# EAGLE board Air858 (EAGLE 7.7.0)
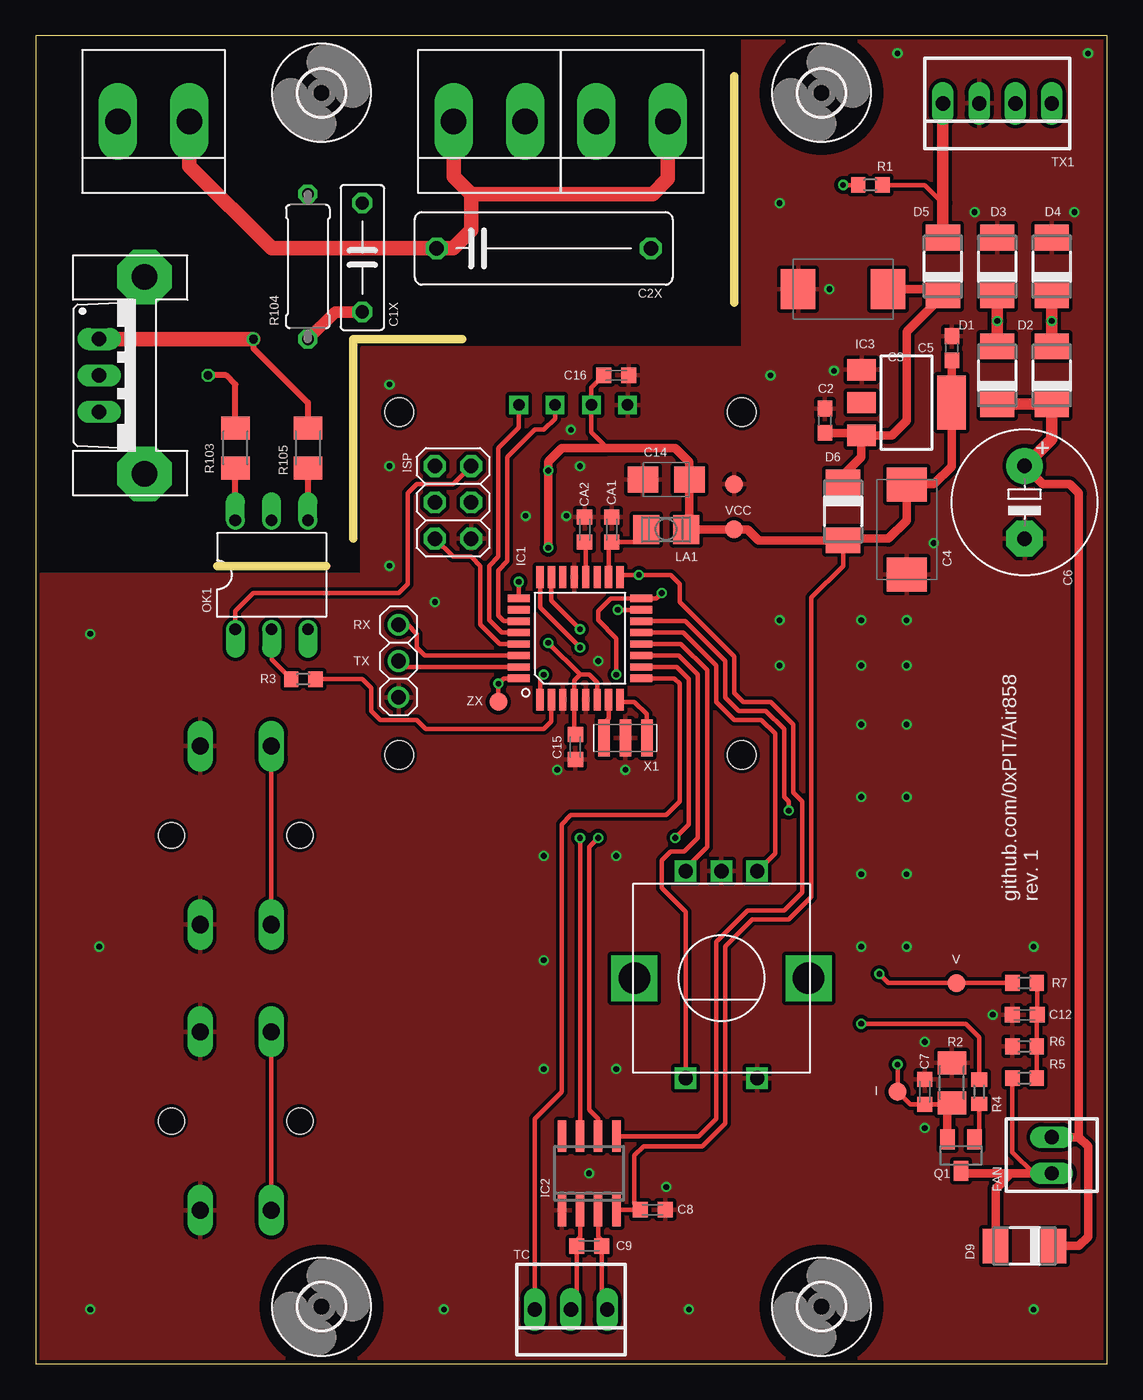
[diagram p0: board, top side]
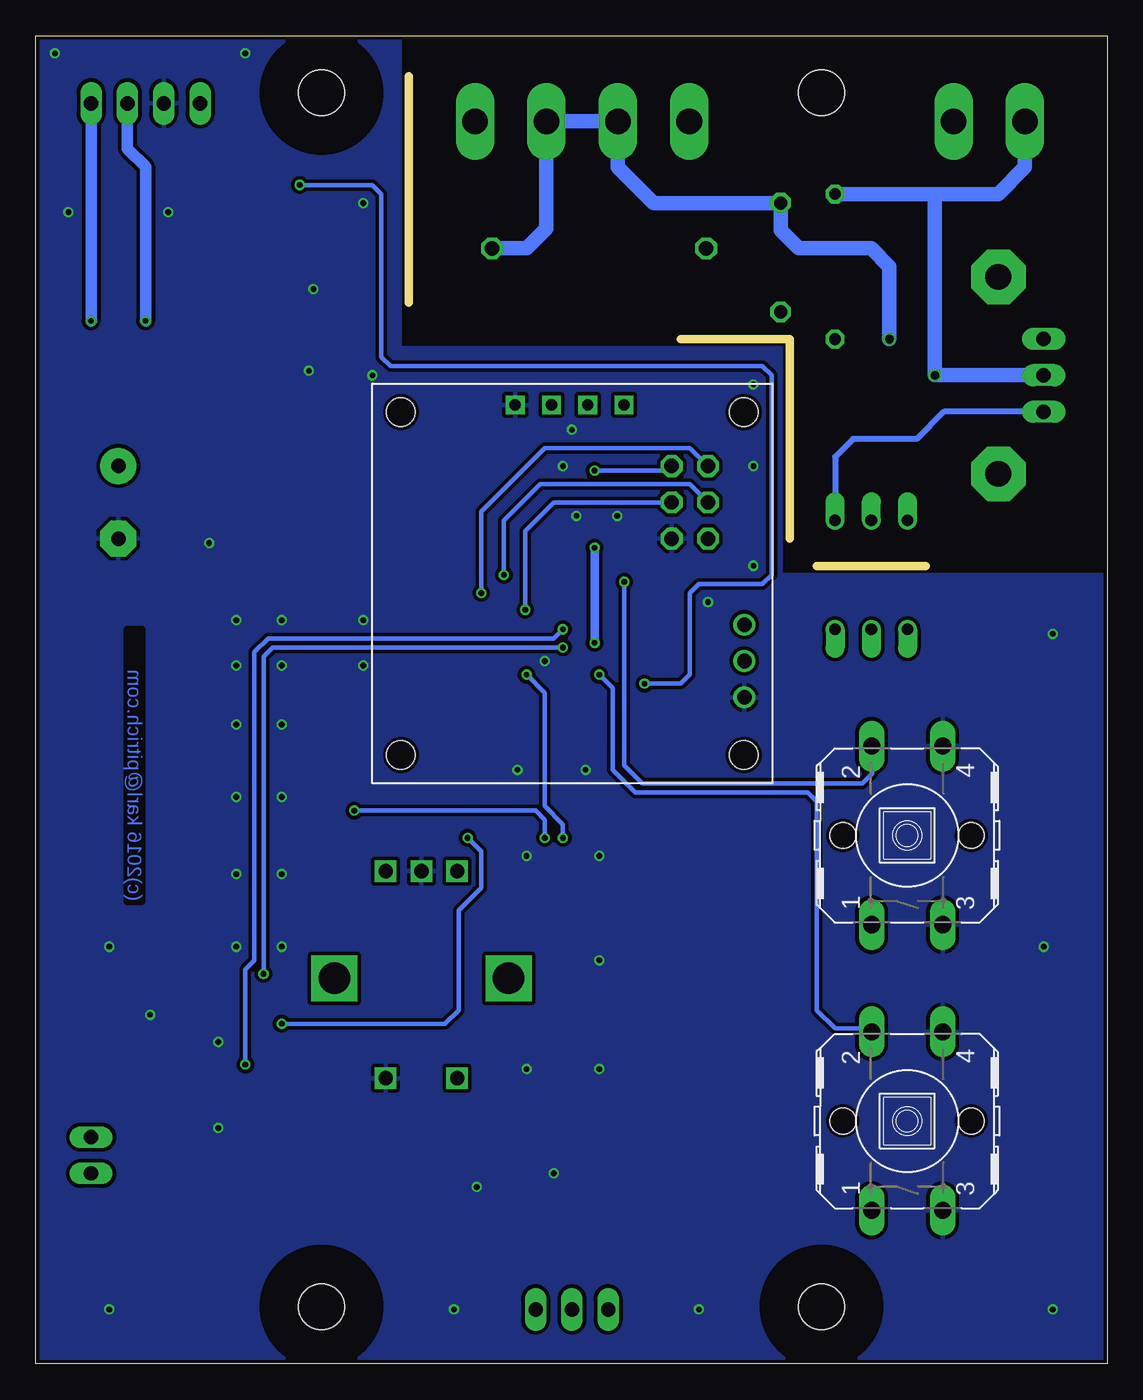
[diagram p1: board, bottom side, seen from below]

Size 75 x 93 mm. Coordinates in mm from the lower left corner, seen from the top.
Outline: 0,0 75,0 75,93 0,93 0,0
Copper layers (1*16): Top 0.035mm / dielectric 1.5mm / Bottom 0.035mm
Design rules "dirt_cheap_dirty_boards.v1": minimum track width 5mil, minimum drill 12mil, track to track 5mil, track to pad 5mil, pad to pad 5mil, via to via 5mil, smd to smd 0mil, copper to edge 10mil, drill to drill 10mil, minimum pad ring 10mil, minimum via ring 6mil, stop-mask expansion 2mil, vias tented up to drill 25mil, thermal gap 10mil
Milling: 4 lines

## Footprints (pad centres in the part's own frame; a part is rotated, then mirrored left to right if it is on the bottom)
B1,27 = smd 1.27 x 1.27: TP 0,0
C075-032X103 = drill 0.914 octagon: 1 -3.81,0; 2 3.81,0
C0603 = smd 1.1 x 1: 1 -0.85,0; 2 0.85,0
C150-054X183 = drill 1.016 octagon: 1 -7.493,0; 2 7.493,0
SMC_E = smd 2.4 x 2.8: + -3.15,0; - 3.15,0
E5-10,5 = drill 1.016 pad 2.54: + -2.54,0 | drill 1.016 pad 2.54 octagon: - 2.54,0
C0603K = smd 1.05 x 1.08: 1 -0.875,0; 2 0.875,0
B/3528-21W = smd 2.15 x 1.8: + 1.625,0; - -1.625,0
DO-214AC = smd 1.8 x 2.4: A 2.025,0; C -2.025,0
22-23-2021 = drill 1 long: 1 -1.27,0; 2 1.27,0
2POL5MM = drill 1.8 long: 1 -2.5,0; 2 2.5,0
QFP32 = smd 0.508 x 1.524: 1 -2.8,-4.293; 2 -2,-4.293; 3 -1.2,-4.293; 4 -0.4,-4.293; 5 0.4,-4.293; 6 1.2,-4.293; 7 2,-4.293; 8 2.8,-4.293; 17 2.8,4.293; 18 2,4.293; 19 1.2,4.293; 20 0.4,4.293; 21 -0.4,4.293; 22 -1.2,4.293; 23 -2,4.293; 24 -2.8,4.293 | smd 1.524 x 0.508: 9 4.293,-2.8; 10 4.293,-2; 11 4.293,-1.2; 12 4.293,-0.4; 13 4.293,0.4; 14 4.293,1.2; 15 4.293,2; 16 4.293,2.8; 25 -4.293,2.8; 26 -4.293,2; 27 -4.293,1.2; 28 -4.293,0.4; 29 -4.293,-0.4; 30 -4.293,-1.2; 31 -4.293,-2; 32 -4.293,-2.8
SOIC8 = smd 0.6 x 2.2: 1 -1.905,-2.6; 2 -0.635,-2.6; 3 0.635,-2.6; 4 1.905,-2.6; 5 1.905,2.6; 6 0.635,2.6; 7 -0.635,2.6; 8 -1.905,2.6
SOT223 = smd 1.5 x 2: 1 -2.3,-3.15; 2 0,-3.15; 3 2.3,-3.15 | smd 3.8 x 2: 4 0,3.15
2X03 = drill 1.016 octagon: 1 -2.54,-1.27; 2 -2.54,1.27; 3 0,-1.27; 4 0,1.27; 5 2.54,-1.27; 6 2.54,1.27
1X03 = drill 1.016: 1 -2.54,0; 2 0,0; 3 2.54,0
L3225P = smd 1.8 x 2: 1 -1.4,0; 2 1.4,0
DIL06 = drill 0.813 offset: 1 -2.54,-3.81; 2 0,-3.81; 3 2.54,-3.81; 4 2.54,3.81; 5 0,3.81; 6 -2.54,3.81
SSD1306-IIC = drill 0.8 square: GND 10,26.5; SCL 15.08,26.5; SDA 17.62,26.5; VCC 12.54,26.5 | hole 2: 2,2; 26,26; 26,2; 2,26
SOT23 = smd 1 x 1.4: 1 -0.95,-1.1; 2 0.95,-1.1; 3 0,1.1
R0603 = smd 1 x 1.1: 1 -0.85,0; 2 0.85,0
M1206 = smd 1.6 x 2: 1 -1.4,0; 2 1.4,0
0309/10 = drill 0.813 octagon: 1 -5.08,0; 2 5.08,0
B3F-40XX = drill 1.194 long: 1 -6.248,2.489; 2 6.248,2.489; 3 -6.248,-2.489; 4 6.248,-2.489 | hole 1.803: 0,-4.496; 0,4.496
ALPS_EC12E_SW = drill 1 square: A -2.5,-7.5; B 2.5,-7.5; C 0,-7.5; D -2.5,7; E 2.5,7 | drill 2.2 square: GND1 -6.1,0; GND2 6.1,0
TO220BV = drill 1.016 long: G 2.54,-2.54; T1 -2.54,-2.54; T2 0,-2.54
22-23-2031 = drill 1 long: 1 -2.54,0; 2 0,0; 3 2.54,0
22-23-2041 = drill 1 long: 1 -3.81,0; 2 -1.27,0; 3 1.27,0; 4 3.81,0
3,2 = hole 3.2: 0,0
HEATSINK17X7.5TO220 = drill 1.8 pad 3.81 octagon: P$1 -6.9,0; P$2 6.9,0
CSTCR6M = smd 0.8 x 2.6: 1 -1.5,0; 2 0,0; 3 1.5,0

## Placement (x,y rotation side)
0V  PTR1B1,27  [B1,27]  48.9,61.59 0 top
C1X  10n  [C075-032X103]  22.86,77.47 270 top
C2  100~n  [C0603]  55.24,66.04 90 top
C2X  100n  [C150-054X183]  35.56,78.11 0 top
C3  220µ  [SMC_E]  56.52,75.25 180 top
C4  220µ  [SMC_E]  60.96,58.42 270 top
C5  100n  [C0603]  64.14,71.12 90 top
C6  470µ  [E5-10,5]  69.22,60.33 270 top
C7  100n  [C0603K]  62.23,19.05 90 top
C8  100n  [C0603K]  43.18,10.79 0 top
C9  100n  [C0603K]  38.73,8.26 180 top
C12  100n  [C0603K]  69.22,24.45 180 top
C14  10µ  [B/3528-21W]  44.13,61.91 0 top
C15  100n  [C0603K]  37.78,43.18 270 top
C16  100n  [C0603K]  40.64,69.22 180 top
CA1  100n  [C0603K]  40.32,58.42 90 top
CA2  100n  [C0603K]  38.42,58.42 270 top
D1  [DO-214AC]  67.31,69.22 90 top
D2  [DO-214AC]  71.12,69.22 90 top
D3  [DO-214AC]  67.31,76.83 90 top
D4  [DO-214AC]  71.12,76.83 90 top
D5  [DO-214AC]  63.5,76.83 90 top
D6  [DO-214AC]  56.52,59.69 270 top
D9  [DO-214AC]  69.22,8.26 180 top
FAN  J1  [22-23-2021]  71.12,14.61 270 top
HEATER  2POL5MM  [2POL5MM]  8.26,87 0 top
I  PTR1B1,27  [B1,27]  60.33,19.05 0 top
IC1  ATMEGA168  [QFP32]  38.1,50.8 0 top
IC2  MAX31855  [SOIC8]  38.73,13.34 0 top
IC3  LD117  [SOT223]  60.96,67.31 270 top
ISP  [2X03]  29.21,60.33 270 top
JP1  [1X03]  25.4,49.21 270 top
LA1  10µ  [L3225P]  44.13,58.42 180 top
MAINS1  2POL5MM  [2POL5MM]  31.75,87 0 top
MAINS2  2POL5MM  [2POL5MM]  41.75,87 0 top
OK1  MOC3041M  [DIL06]  16.51,55.24 0 top
OLED1  [SSD1306-IIC]  51.44,40.64 0 bottom
Q1  TSM3404  [SOT23]  64.77,14.61 180 top
R1  47k  [R0603]  58.42,82.55 180 top
R2  10R  [M1206]  64.14,19.68 270 top
R3  270R  [R0603]  18.73,47.94 180 top
R4  100R  [R0603]  66.04,19.05 270 top
R5  10k  [R0603]  69.22,20 180 top
R6  1k  [R0603]  69.22,22.23 0 top
R7  10k  [R0603]  69.22,26.67 0 top
R103  360R  [M1206]  13.97,64.14 270 top
R104  51R  [0309/10]  19.05,76.83 90 top
R105  330R  [M1206]  19.05,64.14 90 top
S3  [B3F-40XX]  14,37 90 bottom
S4  [B3F-40XX]  14,17 90 bottom
SW1  EC12E_SW  [ALPS_EC12E_SW]  48,27 180 top
T1  BTA16  [TO220BV]  6.99,69.22 270 top
TC  J2  [22-23-2031]  37.47,3.81 180 top
TX1  J4  [22-23-2041]  67.31,88.27 180 top
U$1  [3,2]  20,89 0 top
U$2  [3,2]  55,89 0 top
U$3  [3,2]  20,4 0 top
U$4  [3,2]  55,4 0 top
U$5  HEATSINK17X7.5TO220  [HEATSINK17X7.5TO220]  7.62,69.22 90 top
V  PTR1B1,27  [B1,27]  64.45,26.67 0 top
VCC  PTR1B1,27  [B1,27]  48.9,58.42 0 top
X1  CSTCR6M00G53Z  [CSTCR6M]  41.27,43.81 180 top
ZX  PTR1B1,27  [B1,27]  32.38,46.35 0 top

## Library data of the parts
0V I V VCC ZX = testpad
C1X C2 C2X C3-C9 C12 C14-C16 CA1 CA2 LA1 R1-R7 R103-R105 = rcl
D1-D6 D9 = diode
FAN = con-molex; MF: MOLEX; MPN: 22-23-2021; OC_FARNELL: 1462926; OC_NEWARK: 25C3832
HEATER MAINS1 MAINS2 OLED1 U$5 = pit
IC1 = tidyeagle
IC2 = AlexW-Eagle-Libraries
IC3 = v-reg
ISP = pinhead
JP1 Q1 = adafruit
OK1 = optocoupler; MF: FAIRCHILD SEMICONDUCTOR; MPN: MOC3041M; OC_FARNELL: 1086677; OC_NEWARK: 78K6090
S3 S4 = switch-omron; MF: OMRON COMPONENTS USA; MPN: B3F-4000; OC_FARNELL: 176434; OC_NEWARK: 36K3105
SW1 = switch-alps; MPN: EC12E2424407; OC_FARNELL: 1520813; OC_NEWARK: 74M1068
T1 = triac
TC = con-molex; MF: MOLEX; MPN: 22-23-2031; OC_FARNELL: 1462950; OC_NEWARK: 30C0862
TX1 = con-molex; MF: MOLEX; MPN: 22-23-2041; OC_FARNELL: 1462920; OC_NEWARK: 38C0355
U$1-U$4 = holes
X1 = murata-filter; MPN: CSTCR6M00G53-R0; OC_FARNELL: 1170434; OC_NEWARK: 25M8759

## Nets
10V_AC1: D5.A R1.1 TX1.4
25V_AC1: D1.A D3.C TX1.2
25V_AC2: D2.A D4.C TX1.1
+3V3: C4.+ C5.1 C8.1 C14.+ C15.1 C16.2 D6.A IC1.4 IC1.6 IC2.4 IC3.4 ISP.2 LA1.1 OK1.1 OLED1.VCC VCC.TP
+24V: C6.+ D1.C D2.C D9.C FAN.1
AREF: CA2.2 IC1.20
AVCC: CA1.1 IC1.18 LA1.2
ENC_A: IC1.12 SW1.B
ENC_B: IC1.13 SW1.A
ENC_SW: IC1.11 SW1.E
FAN: IC1.10 R4.1
FAN-: D9.A FAN.2 Q1.3 R5.2
FAN_SENSE_I: C7.1 I.TP IC1.23 Q1.2 R2.2
FAN_SENSE_V: IC1.24 R7.1 V.TP
GND: 0V.TP C2.2 C3.- C4.- C5.2 C6.- C7.2 C8.2 C12.2 C14.- C15.2 C16.1 CA1.2 CA2.1 D3.A D4.A IC1.3 IC1.5 IC1.21 IC2.1 IC3.1 ISP.6 JP1.3 OLED1.GND R2.1 R6.1 S3.3 S3.4 S4.3 S4.4 SW1.C SW1.D TX1.3 X1.2
HEATER: IC1.2 R3.1
HEATER_DRIVE: HEATER.1 R103.1 R104.2 T1.T2
MAINS_L: C2X.1 HEATER.2 MAINS1.1 MAINS2.2
MAINS_N: C1X.1 C2X.2 MAINS1.2 MAINS2.1 R105.2 T1.T1
MISO: IC1.16 IC2.7 ISP.1
MOSI: IC1.15 ISP.4
N$1: C12.1 R5.1 R6.2 R7.2
N$3: OK1.6 R103.2
N$4: C2.1 C3.+ D5.C D6.C IC3.3
N$5: OK1.2 R3.2
N$8: OK1.4 R105.1 T1.G
N$9: C1X.2 R104.1
N$10: IC1.7 X1.3
N$11: Q1.1 R4.2
N$12: IC1.8 X1.1
REED: IC1.9 TC.3
RESET: IC1.29 ISP.5
RXD: IC1.30 JP1.1
SCK: IC1.17 IC2.5 ISP.3
SCL: IC1.27 OLED1.SCL
SDA: IC1.28 OLED1.SDA
SS: IC1.14 IC2.6
SW1: IC1.1 S4.1 S4.2
SW2: IC1.25 S3.1 S3.2
T+: C9.1 IC2.3 TC.1
T-: C9.2 IC2.2 TC.2
TXD: IC1.31 JP1.2
ZEROX: IC1.32 R1.2 ZX.TP

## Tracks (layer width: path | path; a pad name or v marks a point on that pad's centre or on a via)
10V_AC1
  Top 0.305: R1.1 62.23,82.55 63.5,81.28
  Top 0.813: D5.A 63.5,81.28 TX1.4
25V_AC1  (via drill 0.4)
  Top 0.813: D1.A v67.31,73.03 D3.C
  Bottom 0.813: TX1.2 68.58,85.09 67.31,83.82 v67.31,73.03
25V_AC2  (via drill 0.4)
  Top 0.813: D2.A v71.12,73.03 D4.C
  Bottom 0.813: TX1.1 v71.12,73.03
+3V3  (via drill 0.4)
  Top 0.305: C16.2 38.9,68.34 OLED1.VCC 38.9,65.25 40.01,64.14 | ISP.2 29.21,61.59 26.67,61.59 26.04,60.96 26.04,54.61 25.4,53.98 15.24,53.98 13.97,52.7 OK1.1 | C15.1 37.7,44.14 IC1.4 37.7,47.86 38.1,48.26 | IC1.6 39.3,47.7 38.73,48.26 38.1,48.26 | 38.1,48.26 v35.88,50.48 | IC2.4 40.7,10.79 C8.1 41.91,11.19 41.91,14.61 42.55,15.24 46.67,15.24 48.26,16.83 48.26,29.21 50.16,31.11 52.7,31.11 54.29,32.7 54.29,53.66 56.52,55.88 D6.A
  Top 0.61: v35.88,57.15 v35.88,62.55 35.88,63.18 36.83,64.14 40.01,64.14 44.77,64.14 45.76,63.15 C14.+ 45.76,58.65 LA1.1 VCC.TP 49.85,58.42 50.6,57.66 D6.A 56.63,57.78 59.69,57.78 60.96,59.05 C4.+ 60.98,61.59 62.87,61.59 64.11,62.84 IC3.4 64.11,70.25 C5.1
  Bottom 0.305: ISP.2 30.8,62.55 v35.88,62.55
  Bottom 0.61: v35.88,50.48 v35.88,57.15
+24V
  Top 0.61: 73.03,15.88 73.03,60.96 72.39,61.59 70.48,61.59 C6.+ | FAN.1 73.03,15.88 | 73.03,15.88 73.66,15.24 73.66,8.89 73.03,8.26 D9.C
  Top 0.813: D1.C D2.C 71.12,64.77 C6.+
AREF
  Top 0.305: IC1.20 38.5,57.46 CA2.2
AVCC
  Top 0.305: IC1.18 40.1,57.32 CA1.1 42.49,57.55 LA1.2
ENC_A
  Top 0.305: IC1.12 45.17,50.4 46.99,48.58 46.99,36.2 45.5,34.7 SW1.B
ENC_B
  Top 0.305: IC1.13 45.32,51.2 47.62,48.9 47.62,46.35 48.9,45.09 50.8,45.09 51.75,44.13 51.75,35.75 SW1.A
ENC_SW
  Top 0.305: IC1.11 45.02,49.6 46.35,48.26 46.35,36.83 45.4,35.88 44.45,35.88 43.81,35.24 43.81,33.34 45.5,31.65 SW1.E
FAN  (via drill 0.4)
  Top 0.305: IC1.10 44.86,48.8 45.72,47.94 45.72,37.78 v44.77,36.83 | R4.1 66.04,22.86 65.09,23.81 v57.78,23.81
  Bottom 0.305: v44.77,36.83 43.81,35.88 43.81,33.34 45.4,31.75 45.4,24.77 46.35,23.81 v57.78,23.81
FAN-
  Top 0.305: R5.2 68.36,14.82 69.85,13.34
  Top 0.61: FAN.2 69.85,13.34 68.26,13.34 | 68.26,13.34 64.94,13.34 Q1.3 | D9.A 67.19,12.26 68.26,13.34
FAN_SENSE_I  (via drill 0.4)
  Top 0.305: IC1.23 36.1,53.44 v38.1,51.44 | v60.33,20.95 I.TP 61.2,18.18 C7.1 64.05,18.18
  Top 0.61: R2.2 64.05,18.18 63.82,17.95 Q1.2
  Bottom 0.305: v38.1,51.44 38.73,50.8 58.74,50.8 59.69,49.85 59.69,28.26 60.33,27.62 v60.33,20.95
FAN_SENSE_V  (via drill 0.4)
  Top 0.305: IC1.24 35.3,52.97 v38.1,50.16 | v59.05,27.3 59.69,26.67 64.14,26.67 V.TP R7.1
  Bottom 0.305: v38.1,50.16 58.42,50.16 59.05,49.53 v59.05,27.3
GND  (via drill 0.4)
  other vias: 41.27,41.59 36.51,41.59 38.73,13.34 4.45,29.21 52.07,52.07 55.88,69.53 52.07,81.28 52.07,48.9 57.78,48.9 57.78,52.07 60.96,48.9 60.96,44.77 57.78,44.77 40.64,35.56 40.64,20.64 60.96,39.69 60.96,34.29 44.13,12.38 55.56,75.25 65.72,80.64 72.71,80.64 39.37,49.21 62.23,22.54 66.99,24.45 37.15,59.37 38.1,62.87 60.96,52.07 62.23,16.51 45.72,3.81 28.57,3.81 3.81,3.81 69.85,3.81 35.56,20.64 35.56,35.56 35.56,28.26 3.81,51.12 24.77,68.58 24.77,62.87 24.77,55.88 27.94,53.34 60.33,91.76 73.66,91.76 62.87,57.47 69.85,29.21 57.78,39.69 57.78,34.29 57.78,29.21 60.96,29.21 34.29,59.37 37.47,65.41 51.44,69.22
  pour Bottom (isolate 0.254): 0,0 74.93,0 74.93,93.34 49.53,93.34 49.53,71.12 22.86,71.12 22.86,55.24 0,55.24
  pour Top (isolate 0.254): 0,0 74.93,0 74.93,93.34 49.53,93.34 49.53,71.12 22.86,71.12 22.86,55.24 0,55.24
HEATER
  Top 0.305: IC1.2 36.1,44.99 35.56,44.45 27.3,44.45 26.67,45.09 24.13,45.09 23.5,45.72 23.5,47.31 22.86,47.94 R3.1
HEATER_DRIVE  (via drill 0.6)
  Top 0.406: R103.1 13.97,68.58 13.34,69.22 v12.06,69.22
  Bottom 1.016: HEATER.1 5.75,83.78 7.62,81.92 12.06,81.92 | 12.06,81.92 R104.2 | T1.T2 v12.06,69.22 12.06,81.92
MAINS_L
  Top 1.016: MAINS2.2 44.25,82.98 43.18,81.92 30.48,81.92 | 30.48,81.92 30.48,79.38 29.21,78.11 C2X.1 16.51,78.11 10.76,83.86 HEATER.2 | MAINS1.1 29.25,83.14 30.48,81.92
MAINS_N  (via drill 0.6)
  Top 0.406: v15.24,71.75 15.24,71.12 19.05,67.31 R105.2
  Top 1.016: T1.T1 v15.24,71.75
  Bottom 1.016: C2X.2 40.64,78.11 39.25,79.5 MAINS2.1 MAINS1.2 34.25,83.78 31.75,81.28 C1X.1 22.86,79.38 21.59,78.11 16.51,78.11 15.24,76.83 v15.24,71.75
MISO  (via drill 0.4)
  Top 0.305: IC2.7 v38.1,36.83 | v40.64,48.26 40.64,50.8 39.37,52.07 39.37,52.7 40.27,53.6 IC1.16 43.44,53.6 v43.81,53.98
  Bottom 0.305: ISP.1 29.21,64.14 39.37,64.14 43.81,59.69 v43.81,53.98 | v38.1,36.83 38.1,37.78 39.37,39.05 39.37,46.99 v40.64,48.26
MOSI  (via drill 0.4)
  Top 0.305: IC1.15 v40.73,52.8
  Bottom 0.305: v40.73,52.8 40.73,58.33 38.73,60.33 ISP.4
N$1
  Top 0.305: R7.2 70.09,26.64 C12.1 70.06,24.42 R6.2 R5.1
N$3
  Top 0.406: OK1.6 R103.2
N$4
  Top 0.305: 57.63,65.19 IC3.3
  Top 0.61: C2.1 57.63,65.19 | D6.C 56.52,62.23 57.78,63.5 57.78,64.98 IC3.3 59.93,65.01 60.96,66.04 60.96,72.27 D5.C 63.06,75.25 C3.+
N$5
  Top 0.305: R3.2 16.51,49.31 OK1.2
N$8
  Top 0.406: R105.1 OK1.4
  Bottom 0.406: T1.G 11.43,66.67 13.34,64.77 17.78,64.77 19.05,63.5 OK1.4
N$9
  Top 0.813: R104.1 20.95,73.66 C1X.2
N$10
  Top 0.305: X1.3 39.77,44.85 40.1,45.18 IC1.7
N$11
  Top 0.305: Q1.1 66.04,16.02 R4.2
N$12
  Top 0.305: X1.1 42.77,45.49 41.91,46.35 41.05,46.35 IC1.8
REED
  Top 0.305: TC.3 34.92,17.14 36.83,19.05 36.83,37.78 37.47,38.42 44.13,38.42 45.09,39.37 45.09,47.62 44.71,48 IC1.9
RESET
  Top 0.305: IC1.29 32.47,50.4 31.11,51.75 31.11,55.88 30.48,56.52 29.21,56.52 ISP.5
RXD
  Top 0.305: IC1.30 27.23,49.6 26.67,50.16 26.67,51.12 26.04,51.75 JP1.1
SCK  (via drill 0.4)
  Top 0.305: IC1.17 41.05,55.24 v42.23,55.24 44.45,55.24 45.09,54.61 45.09,53.34 48.9,49.53 48.9,46.99 49.53,46.35 51.44,46.35 53.02,44.77 53.02,40.01 53.66,39.37 53.66,33.02 52.39,31.75 49.85,31.75 47.62,29.53 47.62,17.14 46.41,15.94 IC2.5
  Bottom 0.305: ISP.3 29.21,61.59 39.69,61.59 42.23,59.05 v42.23,55.24
SCL
  Top 0.305: IC1.27 32.77,52 32.38,52.39 32.38,55.56 33.02,56.2 33.02,63.5 34.92,65.41 35.56,65.41 36.35,66.2 OLED1.SCL
SDA
  Top 0.305: IC1.28 32.62,51.2 31.75,52.07 31.75,55.88 32.38,56.52 32.38,64.14 33.81,65.56 OLED1.SDA
SS  (via drill 0.4)
  Top 0.305: IC2.6 39.37,17.14 38.73,17.78 38.73,36.2 v39.37,36.83 | IC1.14 45.47,52 48.26,49.21 48.26,46.67 49.21,45.72 51.12,45.72 52.39,44.45 52.39,39.69 52.7,39.37 v52.7,38.73
  Bottom 0.305: v52.7,38.73 40.01,38.73 39.37,38.1 v39.37,36.83
SW1  (via drill 0.4)
  Top 0.305: IC1.1 35.3,48 v35.56,48.26 | S4.2 S4.1
  Bottom 0.305: v35.56,48.26 34.61,47.31 34.61,41.59 33.02,40.01 20.95,40.01 20.32,39.37 20.32,24.77 19.05,23.5 16.74,23.5 S4.2
SW2  (via drill 0.4)
  Top 0.305: S3.2 S3.1 | IC1.25 v33.81,54.76
  Bottom 0.305: S3.2 16.44,41.34 17.14,40.64 32.54,40.64 33.81,41.91 v33.81,54.76
T+
  Top 0.305: IC2.3 39.37,8.89 39.61,8.65 C9.1 39.61,4.21 TC.1
T-
  Top 0.305: IC2.2 38.1,8.89 37.86,8.65 C9.2 37.86,4.21 TC.2
TXD
  Top 0.305: IC1.31 25.81,48.8 JP1.2
ZEROX  (via drill 0.4)
  Top 0.305: R1.2 v56.52,82.55 | IC1.32 32.76,48 v32.38,47.62 ZX.TP
  Bottom 0.305: v56.52,82.55 51.44,82.55 50.8,81.92 50.8,70.48 50.16,69.85 24.13,69.85 23.5,69.22 23.5,55.24 24.13,54.61 28.57,54.61 29.21,53.98 29.21,48.26 29.84,47.62 v32.38,47.62

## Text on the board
Bottom: (c)2016 karl@pitrich.com
tNames: RX | TX | github.com/0xPIT/Air858 / rev. 1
